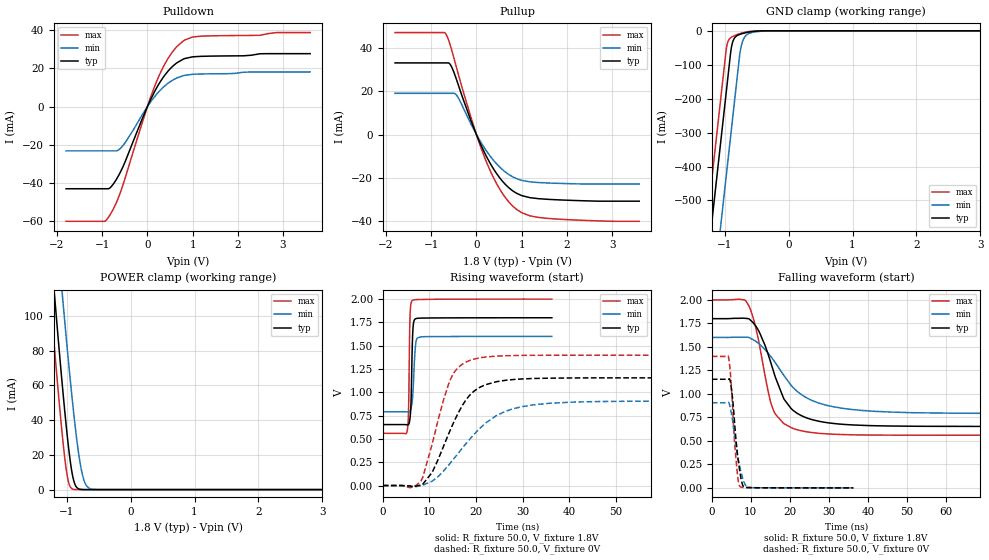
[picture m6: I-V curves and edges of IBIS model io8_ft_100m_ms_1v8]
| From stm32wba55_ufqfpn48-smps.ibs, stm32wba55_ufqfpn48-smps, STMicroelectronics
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[Model]   io8_ft_100m_ms_1v8
Model_type I/O
Polarity   Non-Inverting
Enable   Active-Low
| CAP_THRESHOLD on pad IOFT is "UDTCAPC" :
| Rising=30.0% of vddiom   Falling=70.0% of vddiom
| C_comp min and max val. don't necessarily correlate with the min and max pvt
| but are the smallest and greatest pad capacitance found.
| var   typ   min   max
C_comp   2.20761pF  2.09933pF  2.39591pF
|C_comp_pullup   1.38185pF  1.31775pF  1.46416pF
|C_comp_pulldown   825.76019fF  781.57502fF  931.75609fF
Vinl = 800.0mV
Vinh = 1.0V
Vmeas = 900.0mV   | Reference voltage for timing measurements
Cref  = 50.0pF   | Timing specification test load capacitance value
Rref  = 1.0MOhm   | Timing specification test load resistance value
Vref  = 990.0mV   | Timing specification test load voltage
[Model Spec]
| TIME_THRESHOLD on pin ZIV11 is "CMOS" :
| Rising=50.0% of vdd   Falling=50.0% of vdd
Vinl 702.50000mV 642.50000mV 771.50000mV
Vinh 1.09050V 944.50000mV 1.21950V
| variable   typ   min   max
[Temperature Range] 25.0 140.0 -40.0
| variable   typ   min   max
[Voltage Range] 1.8V 1.6V 2.0V
| variable   typ   min   max
[POWER Clamp Reference] 1.8V 1.6V 2.0V
| variable   typ   min   max
[GND Clamp Reference] 0V 0V 0V
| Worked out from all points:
|   slope of the pulldown table from 0 to 0.27 V, typ, clamps not added: 21.7 ohm
|   slope of the pullup table from 0 to 0.27 V, typ, clamps not added: 22.5 ohm
|   GND clamp passes 1 mA (typ) near -0.51 V on its own axis
|   POWER clamp passes 1 mA (typ) near -0.83 V on its own axis
|   rising waveform, R_fixture 50.0, V_fixture 1.8V: 20-80 % time 321ps typ, 505ps min, 248ps max; typ from 0.654 V to 1.8 V
|   falling waveform, R_fixture 50.0, V_fixture 1.8V: 20-80 % time 6.53ns typ, 10.1ns min, 4.39ns max; typ from 1.8 V to 0.654 V
|   rising waveform, R_fixture 50.0, V_fixture 0V: 20-80 % time 6.49ns typ, 10.2ns min, 4.69ns max; typ from 0 V to 1.16 V
|   falling waveform, R_fixture 50.0, V_fixture 0V: 20-80 % time 1.6ns typ, 2.13ns min, 1.33ns max; typ from 1.16 V to 0 V
[POWER Clamp]
-1.8V     396.4mA    438.1mA    365.5mA
-1.26V    143.5mA    194.6mA    112.6mA
-1.19V    112.3mA    164.2mA    81.56mA
-1.06V    57.23mA    109.3mA    28.68mA
-1.02V    41.75mA    93.06mA    15.5mA
-980mV    27.6mA     77.28mA    5.935mA
-910mV    8.693mA    51.24mA    382.3uA
-850mV    1.642mA    31.41mA    23.97uA
-760mV    69.41uA    9.714mA    358.6nA
-700mV    7.83uA     2.919mA    21.79nA
-620mV    424.6nA    410.3uA    573.9pA
3.6V      0A         0A         0A
[GND Clamp]
-1.8V     -1.583A    -1.83A     -1.456A
-1.43V    -953.9mA   -1.201A    -826.8mA
-1.24V    -630.9mA   -877.8mA   -503.8mA
-1.05V    -307.9mA   -554.8mA   -180.8mA
-970mV    -171.9mA   -418.8mA   -48.31mA
-910mV    -69.87mA   -316.8mA   -20.91mA
-880mV    -36.5mA    -265.8mA   -17.19mA
-830mV    -17.68mA   -180.8mA   -12.97mA
-750mV    -9.66mA    -53.66mA   -7.697mA
-690mV    -6.479mA   -19.19mA   -4.622mA
-600mV    -3.058mA   -6.478mA   -1.59mA
3.6V      1.281nA    1.39uA     517.2pA
| variable   typ   min   max
[Pullup Reference] 1.8V 1.6V 2.0V
| variable   typ   min   max
[Pulldown Reference] 0V 0V 0V
[Pullup]
-1.8V     33.1mA     19.06mA    47.1mA
-680mV    33.1mA     19.06mA    46.54mA
-570mV    32.05mA    19.06mA    40.63mA
-430mV    24.73mA    17.91mA    30.12mA
-120mV    6.338mA    4.782mA    7.854mA
200mV     -9.203mA   -6.891mA   -11.54mA
530mV     -20.35mA   -15.28mA   -25.66mA
690mV     -24.02mA   -18.04mA   -30.41mA
880mV     -26.99mA   -20.26mA   -34.39mA
1.18V     -29.09mA   -21.8mA    -37.49mA
1.56V     -29.85mA   -22.32mA   -38.64mA
3.6V      -30.74mA   -22.8mA    -40.02mA
[Pulldown]
-1.8V     -42.97mA   -23.15mA   -59.99mA
-950mV    -42.97mA   -23.15mA   -59.99mA
-850mV    -42.87mA   -23.15mA   -57.45mA
-670mV    -37.41mA   -23.03mA   -49.3mA
-550mV    -31.91mA   -20.61mA   -41.6mA
10mV      539.8uA    356.7uA    722uA
230mV     10.88mA    7.174mA    14.64mA
500mV     19.69mA    12.93mA    26.79mA
790mV     24.78mA    16.15mA    34.26mA
1V        26.02mA    16.89mA    36.38mA
1.18V     26.27mA    17.05mA    36.82mA
3.6V      27.68mA    18.11mA    38.71mA
[Ramp]
dV/dt_r 693.10678mV/6.45982ns 543.25407mV/10.05085ns 838.8433mV/4.58325ns
dV/dt_f 687.69038mV/6.32917ns 484.93821mV/10.12426ns 864.00217mV/4.33683ns
R_load = 50.0
| Removed startup time: 0s 0s 0s  .
| Removed end time: 36.25ns.
[Rising Waveform]
R_fixture   = 50.0
V_fixture   = 1.8V
V_fixture_min = 1.6V
V_fixture_max = 2.0V
0s        653.8mV    791.8mV    560mV
5.2ns     651.5mV    790.6mV    578.9mV
5.5ns     653.8mV    788.6mV    781.9mV
5.75ns    694.9mV    793.5mV    1.649V
5.85ns    732.7mV    800.3mV    1.841V
6.05ns    900.7mV    828.5mV    1.956V
6.35ns    1.561V     927.9mV    1.987V
6.95ns    1.787V     1.471V     1.994V
7.4ns     1.794V     1.583V     1.995V
36.25ns   1.8V       1.6V       2V
| Removed startup time: 0s 0s 0s  .
| Removed end time: 199.25ns.
[Falling Waveform]
R_fixture   = 50.0
V_fixture   = 1.8V
V_fixture_min = 1.6V
V_fixture_max = 2.0V
0s        1.8V       1.6V       2V
8.6ns     1.803V     1.603V     1.995V
11.1ns    1.73V      1.563V     1.728V
14.35ns   1.429V     1.437V     1.039V
15.85ns   1.231V     1.355V     816.9mV
18.5ns    942.5mV    1.192V     681.6mV
24.2ns    745.3mV    959.2mV    596.6mV
33.7ns    675.4mV    844.4mV    566.7mV
50.65ns   656mV      800.2mV    560.3mV
199.3ns   653.8mV    791.8mV    560mV
| Removed startup time: 0s 0s 0s  .
| Removed end time: 199.2ns.
[Rising Waveform]
R_fixture   = 50.0
V_fixture   = 0V
V_fixture_min = 0V
V_fixture_max = 0V
0s        4.66nV     680.4nV    3.931nV
8.15ns    4.375mV    145.9uV    47.61mV
10.6ns    142.5mV    47.3mV     447.3mV
13.05ns   424.9mV    158.5mV    923.7mV
14.95ns   650.8mV    271mV      1.185V
18.55ns   965mV      491.9mV    1.34V
21.8ns    1.077V     658.8mV    1.377V
28.6ns    1.14V      832.6mV    1.395V
40.65ns   1.154V     894.9mV    1.398V
199.2ns   1.155V     905.4mV    1.398V
| Removed startup time: 0s 0s 0s  .
| Removed end time: 36.25ns.
[Falling Waveform]
R_fixture   = 50.0
V_fixture   = 0V
V_fixture_min = 0V
V_fixture_max = 0V
0s        1.155V     905.5mV    1.398V
4.25ns    1.155V     909.7mV    1.393V
4.65ns    1.146V     865.7mV    1.266V
5.1ns     1.025V     769.2mV    1.003V
6.15ns    522.6mV    451.4mV    320.8mV
6.7ns     311.6mV    312.9mV    90.55mV
7.15ns    176.7mV    224.8mV    17.66mV
8ns       20.46mV    88.64mV    4.134mV
9.65ns    2.711mV    4.075mV    2.225mV
36.25ns   29.96uV    72.04uV    10.49uV
